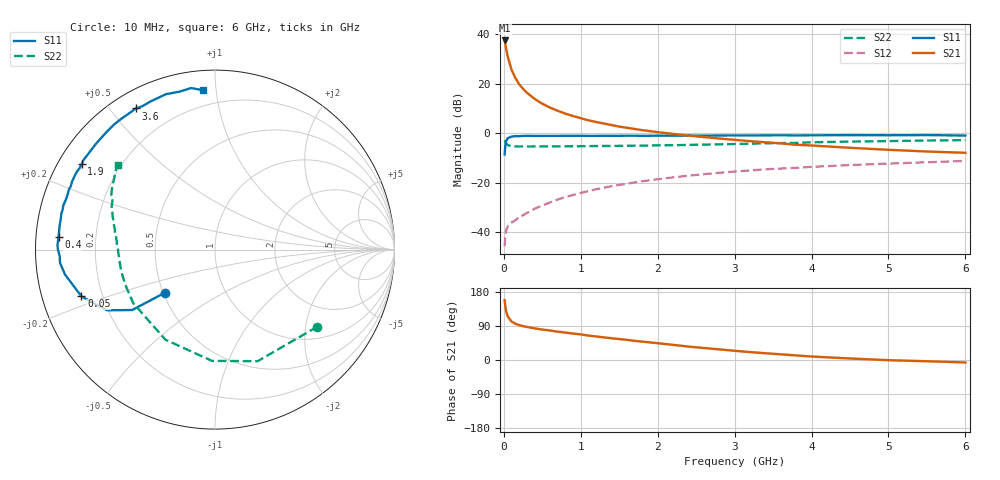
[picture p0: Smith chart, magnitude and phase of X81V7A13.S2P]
! SIEMENS Small Signal Semiconductors
! BFP136W
! Si NPN RF Bipolar Junction Transistor in SOT343
! VCE = 1.75 V  IC = 130 mA
! Common Emitter S-Parameters:  September  1994
# GHz  S  MA  R  50
!  f  S11  S21  S12  S22
! GHz  MAG  ANG  MAG  ANG  MAG  ANG  MAG  ANG
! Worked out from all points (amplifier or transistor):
!   40 points, 10 MHz to 6 GHz, reference 50 ohm
!   highest |S21| = 37.4 dB at 10 MHz (marker M1)
!   |S21| within 3 dB of that: start of sweep to 28.24 MHz
!   unconditionally stable (mu >= 1): 409.8 MHz to 3.024 GHz; 3.759 GHz to 3.851 GHz; 5.924 GHz to end of sweep
!   at 200 MHz: K = 0.78, MSG = 26.8 dB, |S12| = -34.0 dB
!   at 1.5 GHz: K = 1.11, MAG = 9.7 dB, |S12| = -20.9 dB
!   at 6 GHz: K = 1.01, MAG = 1.0 dB, |S12| = -11.3 dB
!   S11 on the Smith chart (normalised r, x): 10 MHz: 0.51, -0.28; 50 MHz: 0.12, -0.17; 400 MHz: 0.07, +0.04; 1.9 GHz: 0.07, +0.29; 3.6 GHz: 0.07, +0.58; 6 GHz: 0.11, +0.92
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0.01  0.3691 -139.3  74.07 158.0  0.0052 65.3  0.7139 -37.0
0.02  0.5713 -143.9  61.9 140.3  0.0085 52.6  0.6655 -69.1
0.03  0.6892 -150.6  50.61 128.5  0.0107 45.9  0.6203 -91.5
0.05  0.7884 -160.7  35.12 115.0  0.0131 37.5  0.573 -118.8
0.1  0.8473 -170.6  19.04 101.6  0.0155 38.2  0.5445 -146.8
0.15  0.8668 -175.1  12.91 95.7  0.0174 42.5  0.5367 -157.7
0.2  0.866 -177.6  9.662 92.0  0.02 45.6  0.5353 -163.5
0.25  0.875 180.0  7.794 89.3  0.0219 49.1  0.5361 -167.2
0.3  0.8782 178.5  6.51 87.2  0.0243 52.8  0.535 -169.7
0.4  0.8747 175.3  4.899 83.5  0.0297 56.3  0.536 -173.0
0.5  0.8747 173.0  3.908 80.3  0.0344 58.8  0.5363 -175.4
0.7  0.8758 168.8  2.814 74.8  0.0455 62.7  0.5396 -178.2
0.9  0.8776 165.4  2.204 69.8  0.0561 63.2  0.5411 179.4
1.1  0.876 161.2  1.807 64.4  0.0674 63.4  0.5448 177.8
1.5  0.8817 154.7  1.351 55.3  0.0897 61.9  0.5506 174.6
1.9  0.8821 147.4  1.093 46.4  0.1115 58.7  0.5609 171.5
2.2  0.885 142.5  0.96 40.0  0.1273 56.0  0.5683 168.9
3.2  0.8967 125.5  0.686 20.9  0.1758 45.7  0.6086 159.9
3.6  0.9019 119.3  0.619 15.0  0.1922 41.7  0.6273 156.3
4.5  0.9081 107.5  0.504 4.0  0.2253 33.0  0.6725 148.4
5.5  0.9097 98.4  0.424 -3.3  0.2574 24.9  0.7063 141.7
6  0.8902 94.2  0.399 -6.5  0.2737 20.5  0.7195 138.8
